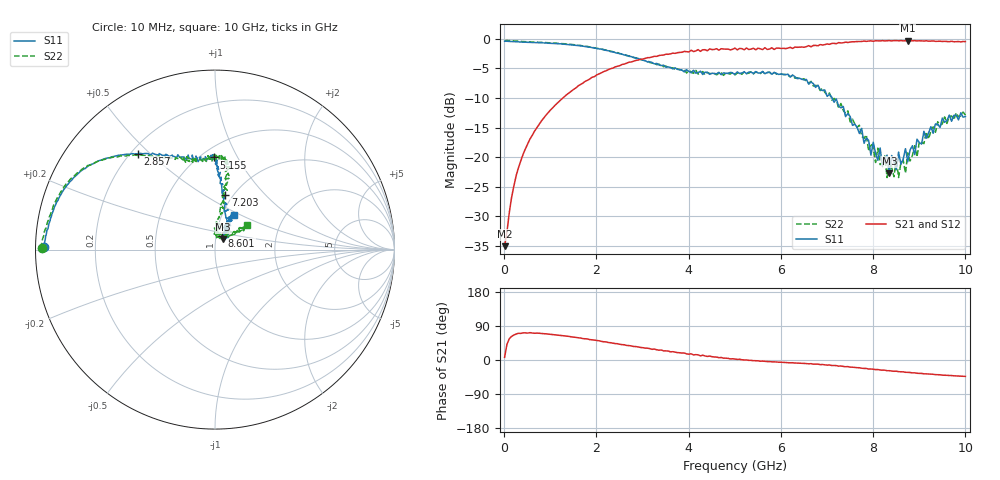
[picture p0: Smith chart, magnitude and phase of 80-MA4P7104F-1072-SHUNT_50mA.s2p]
!Agilent Technologies,E8364C,MY48140145,A.09.42.15
!Agilent E8364C: A.09.42.15
!Date: Wednesday, December 02, 2020 11:08:31
!Correction: S11(Full 2 Port(1,2))
!S21(Full 2 Port(1,2))
!S12(Full 2 Port(1,2))
!S22(Full 2 Port(1,2))
!S2P File: Measurements: S11, S21, S12, S22:
# Hz S  dB  R 50
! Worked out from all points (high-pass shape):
!   201 points, 10 MHz to 10 GHz, reference 50 ohm
!   highest |S21| = -0.30 dB at 8.751 GHz (marker M1); lowest = -35.1 dB at 10 MHz (marker M2)
!   |S21| within 3 dB of the highest: 3.065 GHz to end of sweep
!   lowest |S11| = -22.7 dB at 8.352 GHz (marker M3), VSWR 1.16, Z = 54.5 + j6.19 ohm
!   |S11| at or under -10 dB: 7.11 GHz to end of sweep
!   |S22| runs from -23.5 to -0.3 dB; largest |S21 - S12| = 0.032
!   S11 on the Smith chart (normalised r, x): 10 MHz: 0.02, +0.01; 2.857 GHz: 0.23, +0.46; 5.155 GHz: 0.58, +0.80; 7.203 GHz: 0.92, +0.62; 8.601 GHz: 1.07, +0.17; 10 GHz: 1.14, +0.46
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1e7  -0.42 179.3  -35.06 7.1  -32.34 -18.3  -0.31 179.6
5.995e7  -0.42 178.6  -32.69 41.0  -33.03 41.0  -0.28 178.4
2.5975e8  -0.51 174.5  -23.15 68.5  -23.19 68.3  -0.39 174.1
5.5945e8  -0.60 169.4  -16.95 72.1  -16.98 72.2  -0.53 168.9
1.7083e9  -1.25 149.7  -7.49 56.5  -7.43 56.9  -1.21 150.1
2.85715e9  -3.29 128.7  -3.66 35.5  -3.70 35.0  -3.22 130.2
3.35665e9  -4.44 119.0  -2.83 25.9  -2.92 26.6  -4.30 121.0
5.005e9  -5.98 91.2  -1.57 2.6  -1.50 1.8  -6.13 92.0
5.15485e9  -5.79 90.8  -1.67 0.6  -1.61 0.4  -6.00 89.5
6.7033e9  -7.58 87.8  -1.13 -10.9  -1.09 -10.1  -7.98 81.9
7.2028e9  -10.21 79.4  -0.83 -14.9  -0.80 -15.3  -10.44 82.1
8.05195e9  -19.39 64.2  -0.33 -25.4  -0.35 -24.7  -20.91 80.7
8.25175e9  -20.29 41.5  -0.36 -26.8  -0.36 -27.4  -19.81 87.2
8.3017e9  -19.67 56.1  -0.34 -28.2  -0.30 -27.4  -23.46 82.3
8.35165e9  -22.74 50.8  -0.31 -28.2  -0.35 -28.7  -20.50 72.1
8.4016e9  -19.74 43.3  -0.36 -28.9  -0.31 -29.1  -21.72 87.6
8.55145e9  -19.15 50.5  -0.34 -30.7  -0.28 -30.4  -23.45 75.1
8.6014e9  -21.22 62.5  -0.31 -31.2  -0.34 -31.0  -20.98 55.3
8.7013e9  -18.58 58.2  -0.34 -32.4  -0.29 -31.6  -22.72 53.5
8.75125e9  -20.78 60.9  -0.30 -32.5  -0.35 -32.9  -19.28 52.6
9.1009e9  -15.64 62.0  -0.38 -36.4  -0.33 -35.6  -17.72 36.9
1e10  -13.13 61.2  -0.48 -43.3  -0.48 -43.4  -12.89 37.7
